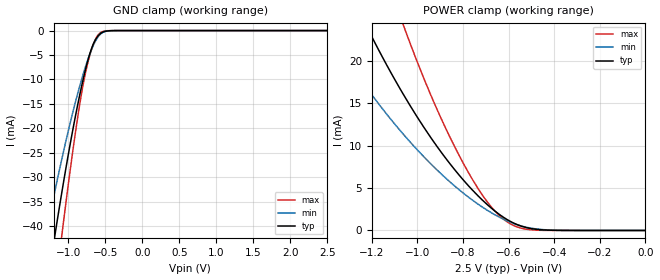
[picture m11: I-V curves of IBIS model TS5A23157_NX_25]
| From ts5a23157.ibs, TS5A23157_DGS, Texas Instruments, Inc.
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[Model]   TS5A23157_NX_25
Model_type  Terminator
| variable   typ   min   max
C_comp   5.96pF   5.33pF   6.40pF
| C_tri-state   5.96pF   5.33pF   6.40pF
[Temperature Range]   40   100   -40
| Ambient temperature   25   85   -40
[Voltage range]   2.5   2.3   2.7
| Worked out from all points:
|   GND clamp passes 1 mA (typ) near -0.59 V on its own axis
|   POWER clamp passes 1 mA (typ) near -0.59 V on its own axis
[GND Clamp]
| TS5A23157_NX_25
|   Voltage   I(typ)   I(min)   I(max)
-2.5V     -195.5mA   -152.1mA   -245.5mA
-1.29V    -52.61mA   -40.86mA   -67.82mA
-1.185V   -42.2mA    -33.07mA   -54.07mA
-1.16V    -39.81mA   -31.28mA   -50.88mA
-1.09V    -33.28mA   -26.41mA   -42.15mA
-1.065V   -31.03mA   -24.73mA   -39.11mA
-885mV    -16.07mA   -13.54mA   -18.92mA
-785mV    -9.053mA   -8.215mA   -9.923mA
-665mV    -2.873mA   -3.151mA   -2.926mA
-560mV    -552.9uA   -666.9uA   -379.4uA
-375mV    -5.824uA   -8.928uA   -871.3nA
2.5V      110.5pA    222.9nA    21.45pA
[POWER Clamp]
| TS5A23157_NX_25
|   Voltage   I(typ)   I(min)   I(max)
-2.5V     126mA      89.26mA    192.8mA
-1.405V   34.6mA     24.07mA    54.1mA
-1.385V   33.36mA    23.22mA    52.12mA
-1.21V    23.34mA    16.33mA    36.02mA
-1.065V   16.18mA    11.43mA    24.42mA
-1.035V   14.83mA    10.51mA    22.24mA
-930mV    10.5mA     7.542mA    15.24mA
-805mV    6.138mA    4.532mA    8.225mA
-710mV    3.448mA    2.662mA    3.966mA
-625mV    1.594mA    1.36mA     1.381mA
-480mV    138.6uA    182.8uA    41.67uA
-31.15fV  110.5pA    790.2pA    25.6pA
